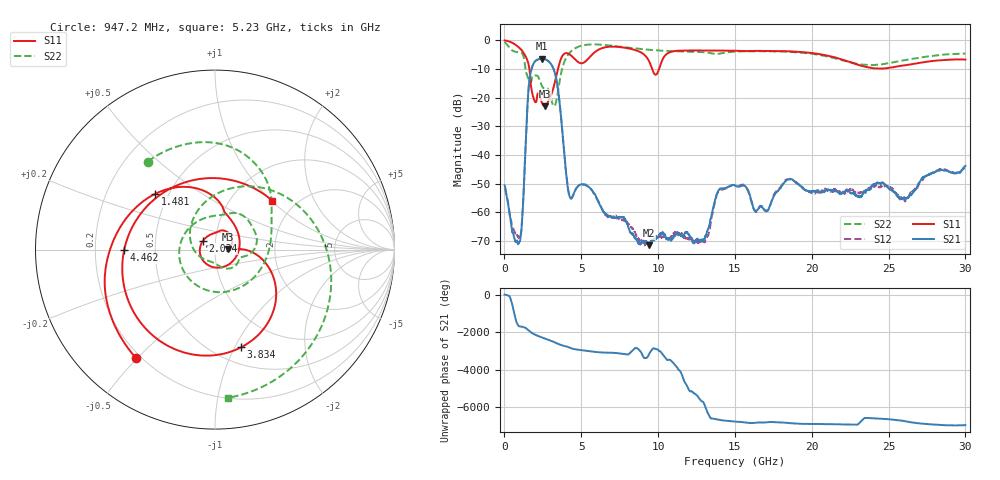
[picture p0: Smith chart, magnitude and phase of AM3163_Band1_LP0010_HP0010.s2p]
!Agilent Technologies,E8364B,MY43040894,A.07.50.67
!Agilent E8364B: A.07.50.67
!Date: Thursday, August 20, 2020 11:17:34
!Correction: S11(Full 2 Port(1,2))
!S21(Full 2 Port(1,2))
!S12(Full 2 Port(1,2))
!S22(Full 2 Port(1,2))
!S2P File: Measurements: S11, S21, S12, S22:
# Hz S  dB  R 50
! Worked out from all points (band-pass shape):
!   3201 points, 10 MHz to 30 GHz, reference 50 ohm
!   highest |S21| = -6.38 dB at 2.428 GHz (marker M1); lowest = -71.4 dB at 9.429 GHz (marker M2)
!   |S21| within 3 dB of the highest: 1.797 GHz to 3.149 GHz (1.351 GHz wide, 54.6 % of centre)
!   lowest |S11| = -23.0 dB at 2.625 GHz (marker M3), VSWR 1.15, Z = 57.6 + j0.401 ohm
!   |S11| at or under -10 dB: 1.622 GHz to 3.483 GHz (1.861 GHz wide, 72.9 % of centre); 9.612 GHz to 10.06 GHz (448.9 MHz wide, 4.56 % of centre)
!   |S22| runs from -23.0 to -0.6 dB; largest |S21 - S12| = 0.0042
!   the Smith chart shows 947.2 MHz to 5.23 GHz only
!   S11 on the Smith chart (normalised r, x): 947.2 MHz: 0.18, -0.50; 1.481 GHz: 0.42, +0.33; 2.034 GHz: 0.87, +0.08; 3.834 GHz: 0.66, -1.06; 4.462 GHz: 0.33, -0.00; 5.23 GHz: 1.53, +1.01
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1e7  -0.06 -8.6  -50.53 3.7  -51.50 18.8  -0.61 -27.6
4.785938e8  -0.78 -62.1  -65.37 -79.8  -64.48 -11.9  -3.42 -148.6
9.471875e8  -2.53 -126.0  -70.47 116.6  -68.76 41.4  -4.19 127.3
1.481384e9  -6.84 136.8  -24.48 -42.7  -24.35 -42.5  -12.34 -78.5
2.034325e9  -21.60 144.7  -7.11 7.7  -7.11 7.7  -12.28 28.7
2.427944e9  -21.60 7.9  -6.38 -122.2  -6.38 -122.3  -15.77 -14.0
2.624753e9  -23.04 2.8  -6.57 179.2  -6.57 179.1  -16.83 -20.4
3.337016e9  -13.29 -5.0  -12.55 -49.4  -12.57 -49.3  -21.95 -137.4
3.833725e9  -4.98 -75.1  -35.76 157.5  -35.69 158.0  -8.43 67.9
4.461641e9  -5.91 -179.7  -54.10 -14.6  -54.19 -15.2  -3.28 -19.7
5.014581e9  -8.01 80.8  -50.19 -83.1  -50.20 -83.3  -1.88 -68.9
5.230134e9  -7.54 40.6  -50.27 -105.3  -50.33 -105.5  -1.64 -85.0
6.382875e9  -2.68 -99.9  -59.12 151.3  -59.43 153.2  -1.57 -153.6
7.591847e9  -2.40 -180.0  -61.56 93.3  -62.43 94.8  -2.27 151.7
9.428734e9  -7.47 82.1  -71.45 91.0  -71.65 90.6  -3.32 80.4
1.000979e10  -10.77 111.9  -68.49 -70.0  -68.18 -122.5  -3.54 59.2
1.238088e10  -3.54 8.2  -70.23 124.1  -69.87 -135.7  -3.98 -21.9
1.5005e10  -3.65 -72.0  -50.60 67.1  -50.54 69.1  -3.93 -90.4
2.000958e10  -4.44 163.6  -52.92 -53.4  -52.70 -56.6  -4.68 136.6
2.276491e10  -8.10 60.2  -53.51 -92.7  -52.76 -95.3  -8.00 21.0
2.500479e10  -9.65 -62.2  -51.52 -167.3  -50.97 -169.9  -7.99 -92.3
3e10  -6.71 110.5  -43.78 -122.5  -44.28 -128.0  -4.61 102.7
